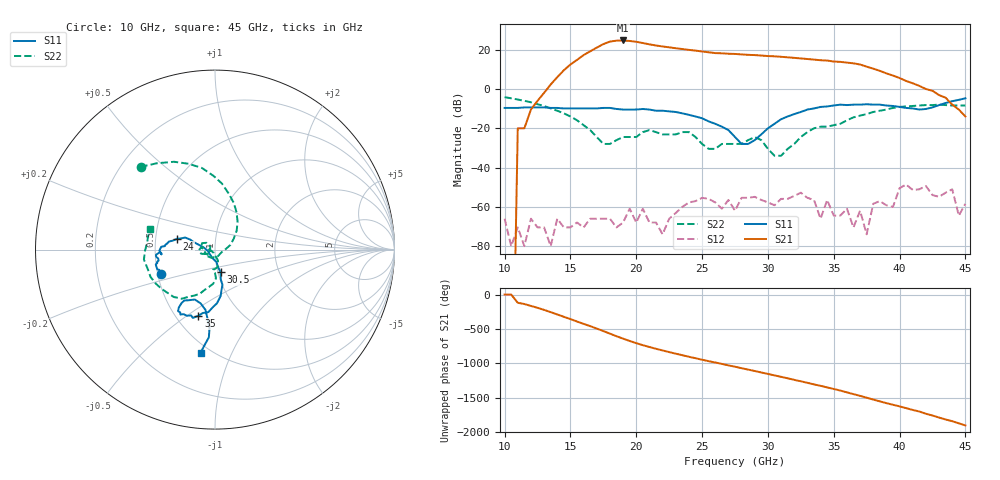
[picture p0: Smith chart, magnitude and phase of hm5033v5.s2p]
! HMMC-5033
! S-PARAMETERS at Vd1 = 3.5V, Id1 = 250mA; Vd2 = 5.0V, Id2 = 450mA.
! LAST UPDATED  03-10-98
#  GHZ  S  MA  R 50
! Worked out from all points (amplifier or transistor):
!   71 points, 10 GHz to 45 GHz, reference 50 ohm
!   highest |S21| = 24.7 dB at 19 GHz (marker M1)
!   |S21| within 3 dB of that: 17.18 GHz to 21.94 GHz (4.763 GHz wide, 24.4 % of centre)
!   unconditionally stable (mu >= 1): start of sweep to end of sweep
!   at 15.5 GHz: K = 198.75, MAG = 15.4 dB, |S12| = -68.0 dB
!   at 27.5 GHz: K = 79.71, MAG = 17.9 dB, |S12| = -61.9 dB
!   at 45 GHz: K = 1182.65, MAG = -11.5 dB, |S12| = -58.4 dB
!   S11 on the Smith chart (normalised r, x): 10 GHz: 0.52, -0.16; 24 GHz: 0.65, +0.08; 30.5 GHz: 1.03, -0.26; 35 GHz: 0.64, -0.56; 45 GHz: 0.44, -0.77
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10  0.33 -156.0  0 -23.0  0.0005 67.0  0.62 132.0
14.5  0.32 -169.0  3 36.0  0.0003 -130.0  0.24 60.0
16  0.32 -169.0  7.3 -67.0  0.0003 -151.0  0.12 30.0
17  0.32 -171.0  11.3 -135.0  0.0005 143.0  0.06 3.0
18  0.33 -175.0  16.1 151.0  0.0005 98.0  0.04 -66.0
18.5  0.31 -177.0  17 113.0  0.0003 110.0  0.05 -113.0
19  0.3 -176.0  17.2 78.0  0.0004 105.0  0.06 -146.0
20  0.3 -176.0  15.9 12.0  0.0004 147.0  0.06 -156.0
21  0.3 177.0  13.7 -44.0  0.0004 108.0  0.09 -178.0
22  0.28 175.0  12.1 -94.0  0.0002 -116.0  0.07 168.0
23  0.26 170.0  10.9 -141.0  0.0007 105.0  0.07 175.0
24  0.22 164.0  9.9 174.0  0.0013 131.0  0.08 153.0
25.5  0.15 158.0  8.6 110.0  0.0016 64.0  0.03 150.0
27.5  0.06 171.0  7.8 29.0  0.0008 24.0  0.04 -160.0
29  0.05 -106.0  7.3 -33.0  0.0018 4.0  0.06 -164.0
30.5  0.13 -76.0  6.8 -97.0  0.0011 3.0  0.02 -153.0
32  0.23 -81.0  6.2 -162.0  0.0019 -54.0  0.04 -83.0
33.5  0.32 -92.0  5.6 132.0  0.0015 155.0  0.1 -83.0
35  0.38 -104.0  5 65.0  0.0006 96.0  0.12 -93.0
37.5  0.41 -118.0  3.7 -62.0  0.0002 128.0  0.23 -104.0
39.5  0.37 -122.0  2.2 -165.0  0.001 71.0  0.33 -124.0
45  0.58 -98.0  0.2 -106.0  0.0012 176.0  0.38 162.0
